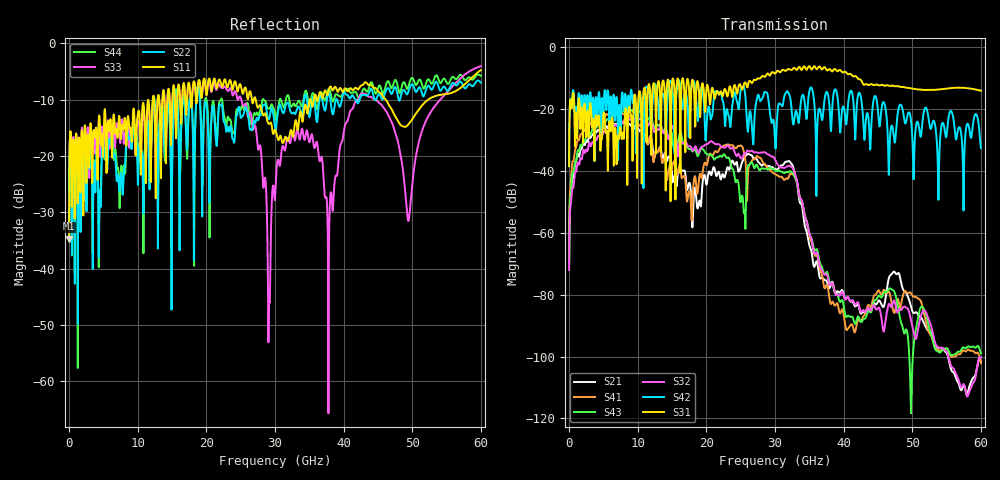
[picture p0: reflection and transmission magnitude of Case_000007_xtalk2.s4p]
! Info: Touchstone file created by circ.  Input file=CasetestDOE_NRZ_template_000007.circ
# Hz S RI R 50
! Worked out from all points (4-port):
!   6000 points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, 10 MHz to 60 GHz, reference 50 ohm
!   strongest paths, dB at 10 MHz, 15.01 GHz, 30.01 GHz, 45.01 GHz, 60 GHz:
!     S31: -38.5, -11.3, -8.6, -12.3, -14.1
!     S42: -38.5, -13.1, -30.5, -20.6, -32.6
!     S32: -72.1, -25.7, -36.3, -84.3, -100.4
!     S43: -69.5, -28.4, -39.8, -80.6, -99.0
!     S41: -66.7, -38.9, -41.0, -78.7, -102.1
!     S21: -69.9, -41.6, -39.4, -82.2, -101.6
!   lowest |S11| = -34.7 dB at 10 MHz (marker M1), VSWR 1.04, Z = 51.2 + j1.43 ohm
!   |S11| at or under -10 dB: start of sweep to 12.19 GHz; 27.2 GHz to 35.08 GHz (7.881 GHz wide, 25.3 % of centre); 46.15 GHz to 52.33 GHz (6.179 GHz wide, 12.5 % of centre)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
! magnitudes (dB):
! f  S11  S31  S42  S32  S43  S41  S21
! 10 MHz  -34.7  -38.5  -38.5  -72.1  -69.5  -66.7  -69.9
! 1.88 GHz  -15.5  -19.9  -16.0  -36.0  -31.8  -28.0  -32.7
! 9.91 GHz  -13.8  -38.0  -21.9  -22.9  -20.2  -23.9  -25.7
! 24.95 GHz  -7.3  -12.2  -14.7  -35.7  -50.0  -31.8  -39.3
! 29.15 GHz  -14.3  -9.1  -19.2  -34.8  -39.1  -39.5  -38.4
! 38.99 GHz  -8.2  -7.6  -14.6  -80.0  -79.7  -82.8  -79.2
! 60 GHz  -4.8  -14.1  -32.6  -100.4  -99.0  -102.1  -101.6
